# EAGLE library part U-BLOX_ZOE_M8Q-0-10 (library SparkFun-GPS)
UBLOX ZOE-M8Q-0-10 u-blox ZOE-M8 standard precision GNSS SiP (System in Package) modules feature the high performance u-blox M8 GNSS engine. ZOE-M8’s ultra-miniature form factor integrates a complete GNSS receiver including SAW filter, LNA and TCXO. Handles all GNSS systems and can simultaneously use up to three of them, with accuracy ranging from 2.5m to 4m. GPS GLONASS BeiDou Galileo This can be corrected with the SBAS or QZSS augmentation systems.
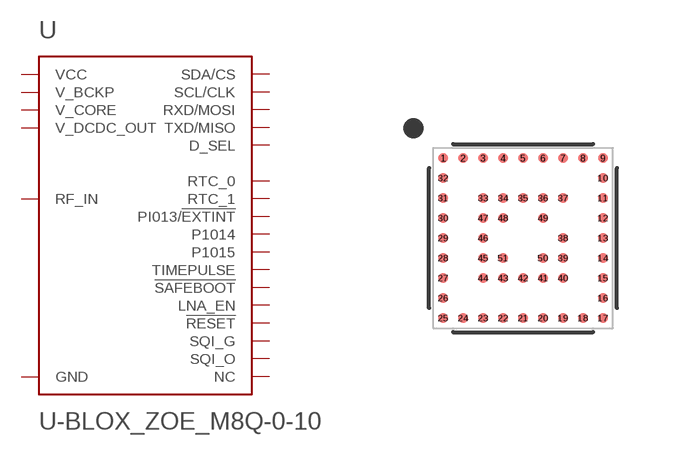
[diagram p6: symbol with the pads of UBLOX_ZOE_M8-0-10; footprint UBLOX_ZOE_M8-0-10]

Designator prefix U

## U-BLOX_ZOE_M8Q-0-10 (PROD_ID: IC-14251)  [UBLOX_ZOE_M8-0-10]
1  GND  pwr
2  SDA/CS
3  GND  pwr
4  RF_IN
5  GND  pwr
6  NC  nc
7  GND  pwr
8  GND  pwr
9  GND  pwr
10  GND  pwr
11  GND  pwr
12  GND  pwr
13  NC  nc
14  NC  nc
15  NC  nc
16  V_BCKP  pwr
17  GND  pwr
18  RTC_0
19  RTC_1
20  !RESET
21  TXD/MISO
22  RXD/MOSI
23  GND  pwr
24  VCC  pwr
25  VCC  pwr
26  V_DCDC_OUT  pwr
27  V_CORE  pwr
28  NC  nc
29  SQI_G
30  SQI_O  nc
31  SQI_G
32  SCL/CLK
33  TIMEPULSE
34  !SAFEBOOT
35  LNA_EN
36  P1015
37  GND  pwr
38  GND  pwr
39  GND  pwr
40  GND  pwr
41  GND  pwr
42  NC  nc
43  PI013/!EXTINT
44  GND  pwr
45  SQI_O  nc
46  SQI_G
47  SQI_G
48  D_SEL
49  GND  pwr
50  P1014
51  NC  nc

## Footprint UBLOX_ZOE_M8-0-10 (pad centres in mm)
UBLOX ZOE-M8Q-0-10 The ZOE-M8G and ZOE-M8Q are u-blox’s super small, highly integrated GNSS SiP (System in Package) modules based on the high performing u-blox M8 concurrent positioning engine. The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
smd 0.25 x 0.25: 1 -1.996,2.004; 2 -1.496,2.004; 3 -0.996,2.004; 4 -0.496,2.004; 5 0.004,2.004; 6 0.504,2.004; 7 1.004,2.004; 8 1.504,2.004; 9 2.004,2.004; 10 2.004,1.504; 11 2.004,1.004; 12 2.004,0.504; 13 2.004,0.004; 14 2.004,-0.496; 15 2.004,-0.996; 16 2.004,-1.496; 17 2.004,-1.996; 18 1.504,-1.996; 19 1.004,-1.996; 20 0.504,-1.996; 21 0.004,-1.996; 22 -0.496,-1.996; 23 -0.996,-1.996; 24 -1.496,-1.996; 25 -1.996,-1.996; 26 -1.996,-1.496; 27 -1.996,-0.996; 28 -1.996,-0.496; 29 -1.996,0.004; 30 -1.996,0.504; 31 -1.996,1.004; 32 -1.996,1.504; 33 -0.996,1.004; 34 -0.496,1.004; 35 0.004,1.004; 36 0.504,1.004; 37 1.004,1.004; 38 1.004,0.004; 39 1.004,-0.496; 40 1.004,-0.996; 41 0.504,-0.996; 42 0.004,-0.996; 43 -0.496,-0.996; 44 -0.996,-0.996; 45 -0.996,-0.496; 46 -0.996,0.004; 47 -0.996,0.504; 48 -0.496,0.504; 49 0.504,0.504; 50 0.504,-0.496; 51 -0.496,-0.496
